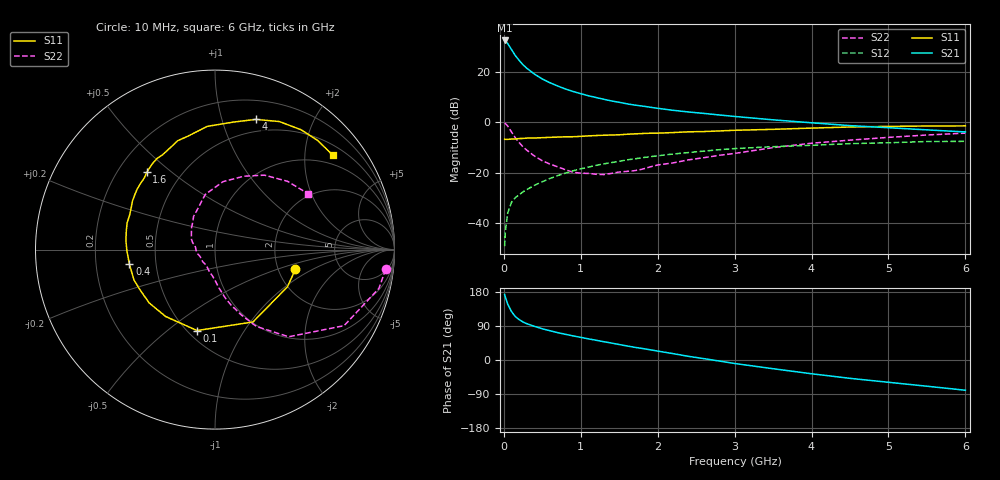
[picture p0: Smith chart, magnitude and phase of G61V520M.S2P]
! SIEMENS Small Signal Semiconductors
! BFG193
! Si NPN RF Bipolar Junction Transistor in SOT223
! VCE = 1.5 V  IC = 20 mA
! Common Emitter S-Parameters:  August  1996
# GHz  S  MA  R  50
!  f  S11  S21  S12  S22
! GHz  MAG  ANG  MAG  ANG  MAG  ANG  MAG  ANG
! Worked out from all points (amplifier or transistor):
!   36 points, 10 MHz to 6 GHz, reference 50 ohm
!   highest |S21| = 32.3 dB at 10 MHz (marker M1)
!   |S21| within 3 dB of that: start of sweep to 87.05 MHz
!   unconditionally stable (mu >= 1): 656.3 MHz to 2.772 GHz
!   at 250 MHz: K = 0.76, MSG = 25.1 dB, |S12| = -27.6 dB
!   at 1.4 GHz: K = 1.06, MAG = 10.7 dB, |S12| = -16.0 dB
!   at 6 GHz: K = 0.94, MSG = 1.9 dB, |S12| = -7.6 dB
!   S11 on the Smith chart (normalised r, x): 10 MHz: 2.48, -0.69; 100 MHz: 0.56, -0.64; 400 MHz: 0.35, -0.07; 1.6 GHz: 0.32, +0.41; 4 GHz: 0.38, +1.29; 6 GHz: 0.74, +2.66
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0.01  0.4612 -13.8  41.24 172.7  0.0035 90.8  0.957 -6.6
0.02  0.4538 -27.2  40.55 166.4  0.0069 80.0  0.9387 -13.3
0.05  0.4553 -62.3  35.83 147.5  0.0158 68.9  0.8349 -30.5
0.1  0.4619 -102.5  27.18 127.8  0.0259 60.2  0.6359 -49.8
0.15  0.4633 -126.5  20.61 114.4  0.032 55.2  0.4864 -61.7
0.2  0.472 -141.0  16.54 106.5  0.0367 55.6  0.3921 -68.1
0.25  0.4742 -151.8  13.59 100.2  0.0417 56.0  0.3213 -73.9
0.3  0.482 -159.4  11.57 95.7  0.0463 56.7  0.2768 -77.9
0.4  0.4838 -170.3  8.854 88.7  0.0563 57.8  0.2115 -84.5
0.5  0.4912 -179.3  7.13 82.3  0.0659 57.9  0.1715 -89.9
0.6  0.4988 174.2  5.999 77.2  0.0766 58.0  0.1473 -95.5
0.7  0.5048 168.3  5.172 72.2  0.0873 57.5  0.1301 -102.7
0.9  0.5128 158.2  4.033 63.6  0.1085 55.1  0.1018 -117.2
1.1  0.533 149.8  3.316 55.8  0.1284 52.1  0.0964 -135.1
1.6  0.5744 131.4  2.297 37.1  0.1784 42.3  0.1058 -178.1
2.2  0.6203 113.6  1.71 16.8  0.2332 29.0  0.1556 147.8
2.8  0.6672 98.1  1.382 -2.7  0.284 15.2  0.2201 122.8
3.5  0.7181 81.7  1.108 -23.0  0.326 -2.1  0.3122 100.0
4  0.7603 72.6  0.968 -36.3  0.347 -11.7  0.3815 83.2
4.5  0.7985 63.3  0.851 -48.4  0.3741 -21.6  0.4389 68.6
5.5  0.8351 46.7  0.701 -69.2  0.4125 -44.3  0.555 43.3
6  0.8408 38.8  0.638 -79.8  0.4151 -57.3  0.6041 31.1
